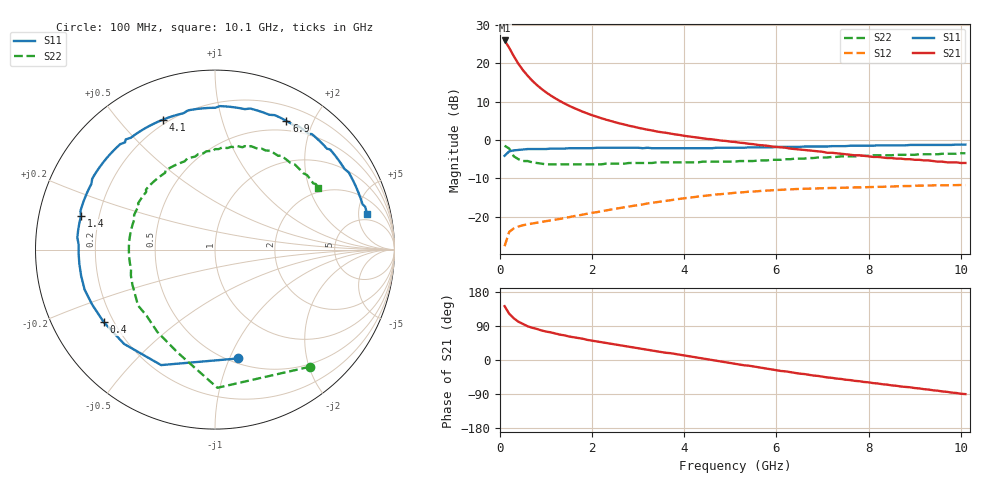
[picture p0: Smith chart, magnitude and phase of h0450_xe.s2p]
!HBFP-0450
!S and NOISE PARAMETERS at Vce=0.5V  Ic=15mA.  LAST UPDATED  09-04-98
# GHZ S MA R  50
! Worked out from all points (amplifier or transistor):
!   101 points, 100 MHz to 10.1 GHz, reference 50 ohm
!   highest |S21| = 26.0 dB at 100 MHz (marker M1)
!   |S21| within 3 dB of that: start of sweep to 248.9 MHz
!   unconditionally stable (mu >= 1): 2.533 GHz to end of sweep
!   at 1.7 GHz: K = 0.85, MSG = 13.8 dB, |S12| = -19.7 dB
!   at 5.1 GHz: K = 1.13, MAG = 4.4 dB, |S12| = -13.8 dB
!   at 10.1 GHz: K = 1.10, MAG = 1.0 dB, |S12| = -11.8 dB
!   lowest NFmin = 1.21 dB at 1.8 GHz
!   S11 on the Smith chart (normalised r, x): 100 MHz: 0.55, -1.08; 400 MHz: 0.16, -0.29; 1.4 GHz: 0.13, +0.12; 4.1 GHz: 0.18, +0.66; 6.9 GHz: 0.37, +1.63; 10.1 GHz: 3.95, +6.36
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0.1  0.62 -78.0  19.89 142.0  0.041 58.0  0.84 -51.0
0.2  0.71 -115.0  15.94 122.0  0.063 43.0  0.77 -89.0
0.3  0.73 -134.0  12.37 110.0  0.07 32.0  0.61 -110.0
0.4  0.74 -147.0  9.85 101.0  0.074 27.0  0.56 -125.0
0.5  0.75 -156.0  8.12 95.0  0.077 25.0  0.53 -136.0
0.6  0.76 -163.0  6.89 89.0  0.079 23.0  0.53 -144.0
0.7  0.76 -169.0  5.93 85.0  0.081 22.0  0.51 -151.0
0.8  0.76 -174.0  5.21 82.0  0.083 22.0  0.5 -157.0
0.9  0.76 -178.0  4.64 78.0  0.085 22.0  0.49 -163.0
1  0.76 178.0  4.18 75.0  0.087 22.0  0.48 -167.0
1.2  0.77 172.0  3.49 70.0  0.091 22.0  0.48 -175.0
1.4  0.77 166.0  2.99 65.0  0.096 23.0  0.48 178.0
1.8  0.78 156.0  2.33 56.0  0.106 22.0  0.48 168.0
2  0.78 152.0  2.1 51.0  0.112 22.0  0.48 163.0
2.5  0.79 142.0  1.7 41.0  0.126 20.0  0.49 154.0
3.5  0.78 123.0  1.26 21.0  0.157 13.0  0.51 137.0
4.1  0.78 112.0  1.11 10.0  0.176 6.0  0.51 127.0
5.1  0.79 93.0  0.94 -10.0  0.204 -7.0  0.52 109.0
6.8  0.82 63.0  0.72 -41.0  0.232 -30.0  0.58 80.0
6.9  0.82 61.0  0.71 -42.0  0.233 -32.0  0.59 78.0
8.5  0.85 36.0  0.58 -67.0  0.246 -52.0  0.63 56.0
10.1  0.87 13.0  0.5 -90.0  0.257 -74.0  0.67 31.0
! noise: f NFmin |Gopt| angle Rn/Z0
1.8  1.21  0.54  -171  0.04
2  1.27  0.55  -167  0.05
2.5  1.39  0.58  -153  0.08
3.5  1.66  0.63  -134  0.18
4  1.82  0.66  -122  0.3
5  2.09  0.7  -101  0.6
5.5  2.24  0.72  -91  0.86
7  2.64  0.76  -62  1.84
8  2.91  0.78  -45  2.55
10  3.45  0.78  -16  4.13
